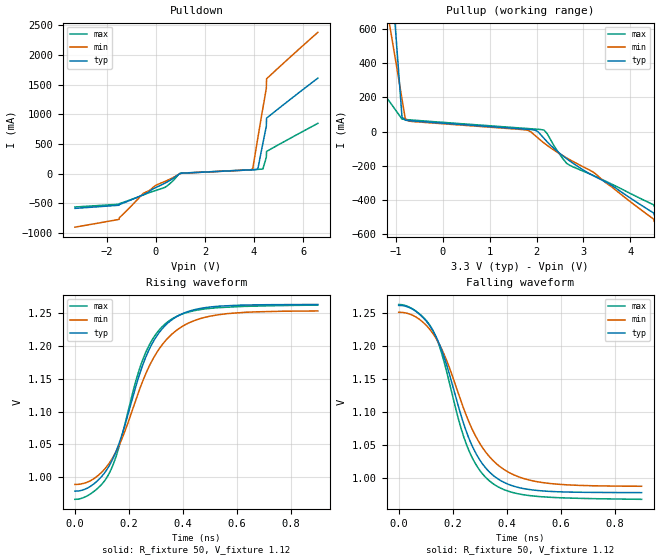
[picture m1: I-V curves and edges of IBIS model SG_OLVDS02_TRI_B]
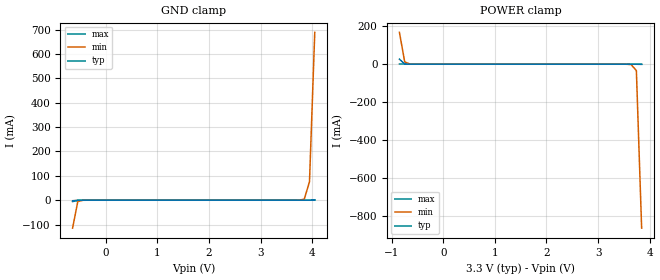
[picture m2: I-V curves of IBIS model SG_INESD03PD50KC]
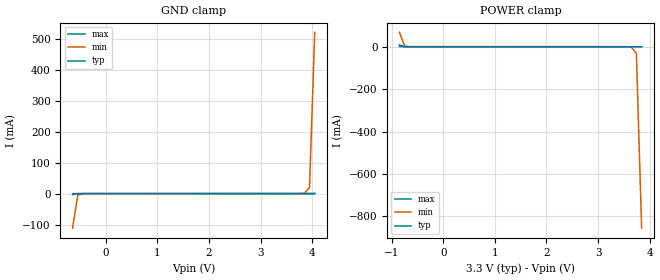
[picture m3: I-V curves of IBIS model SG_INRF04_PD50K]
|   This file is an IBIS representation of the   |
|   Integrated Device Technology, Inc.   |
|   854S54I-02   |
|   DUAL 2:1 AND 1:2, DIFFERENTIAL-TO-LVDS MULTIPLEXER   |
[IBIS Ver]   4.1
[File name]   854s54i_02_3v3.ibs
[File Rev]   1.0
[Date]   16 Apr 2010
[Source]   Originated at Integrated Device Technology, Inc.
[Disclaimer]
IDT hereby grants the user of this IBIS model a non-exclusive,
nontransferable license to use this IBIS model under the following terms.
Before using this IBIS model, the user should read this license.
If the user does not accept these terms,  the IBIS model should be
returned to IDT within 30 days.
   The user is granted this license only to use the IBIS model and
is not granted rights to sell, load, rent, lease or license the IBIS
model in whole or in part, or in modified form to anyone other than
user. User may modify the IBIS model to suit its specific
applications but rights to derivative works and such modifications
shall belong to IDT.
   This IBIS model is provided on an "AS IS" basis and IDT makes
absolutely no warranty with respect to the information contained
herein. IDT DISCLAIMS AND CUSTOMER WAIVES ALL WARRANTIES, EXPRESS
OR IMPLIED, INCLUDING WARRANTIES OF MERCHANTABILITY OR FITNESS FOR
A PARTICULAR PURPOSE. The entire risk as to quality and performance
is with the Customer. ACCORDINGLY, IN NO EVENT SHALL THE COMPANY BE
LIABLE FOR ANY DAMAGES, WHETHER IN CONTRACT OR TORT,INCLUDING ANY
LOST PROFITS OR OTHER INCIDENTAL, CONSEQUENTIAL, EXEMPLARY, OR
PUNITIVE DAMAGES ARISING OUT OF THE USE OR APPLICATION OF THE IBIS
model provided in this package. Further, IDT reserves the right to
make changes without notice to any product herein to improve
reliability, function, or design. IDT does not convey any license
under patent rights or any other intellectual property rights,
including those of third parties.
   IDT is not obligated to provide maintenance or support
for the licensed IBIS model.
[Copyright]   Copyright 2007 by Integrated Device Technology, Inc.
[Component]   854S54KI-02
[Manufacturer] Integrated Device Technology, Inc.
[Package]
|VFQFN 24 Lead
|   typ   min   max
R_pkg   53.3006m   39.9458m   67.5454m
L_pkg   0.925n   0.5704n   1.2967n
C_pkg   0.1079p   0.0821p   0.1352p
[Pin] signal_name  model_name   R_pin   L_pin   C_pin
1   VDD   POWER   67.5454m   1.2967n   0.1352p
2   QA0   SG_OLVDS02_TRI_B   53.7456m   0.9336n   0.1086p
3   nQA0   SG_OLVDS02_TRI_B   39.9458m   0.5704n   0.0821p
4   GND   GND   39.9458m   0.5704n   0.0821p
5   SEL_QB   SG_INESD03PD50KC   53.7456m   0.9336n   0.1086p
6   NC   NC   67.5454m   1.2967n   0.1352p
7   NC   NC   67.5454m   1.2967n   0.1352p
8   INA0   SG_INRF04_PD50K   53.7456m   0.9336n   0.1086p
9   nINA0   SG_INRF04_PMID50   39.9458m   0.5704n   0.0821p
10   INA1   SG_INRF04_PD50K   39.9458m   0.5704n   0.0821p
11   nINA1   SG_INRF04_PMID50   53.7456m   0.9336n   0.1086p
12   NC   NC   67.5454m   1.2967n   0.1352p
13   NC   NC   67.5454m   1.2967n   0.1352p
14   MODE_QAX   SG_INESD03_PD50K   53.7456m   0.9336n   0.1086p
15   GND   GND   39.9458m   0.5704n   0.0821p
16   nQA1   SG_OLVDS02_TRI_B   39.9458m   0.5704n   0.0821p
17   QA1   SG_OLVDS02_TRI_B   53.7456m   0.9336n   0.1086p
18   VDD   POWER   67.5454m   1.2967n   0.1352p
19   NC   NC   67.5454m   1.2967n   0.1352p
20   nINB   SG_INRF04_PD50K   53.7456m   0.9336n   0.1086p
21   INB   SG_INRF04_PMID50   39.9458m   0.5704n   0.0821p
22   nQB   SG_OLVDS02_TRI_B   39.9458m   0.5704n   0.0821p
23   QB   SG_OLVDS02_TRI_B   53.7456m   0.9336n   0.1086p
24   NC   NC   67.5454m   1.2967n   0.1352p
[Diff Pin]  inv_pin  vdiff tdelay_typ tdelay_min  tdelay_max
2   3   NA   0   0   0
8   9   0.15   NA   NA   NA
10   11   0.15   NA   NA   NA
17   16   NA   0   0   0
21   20   0.15   NA   NA   NA
23   22   NA   0   0   0
| Models and submodels in the file (5): SG_OLVDS02_TRI_B (Output), SG_INESD03PD50KC (Input), SG_INRF04_PD50K (Input), SG_INRF04_PMID50 (Input), SG_INESD03_PD50K (Input)
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[Model]   SG_OLVDS02_TRI_B
Model_type   Output
Polarity   Non-Inverting
|   typ   min   max
C_comp   2pF   1.5pF   2.5pF
Vmeas = 1.12V
Rref = 50
Cref = 0
Vref = 1.12V
|   typ   min   max
[Voltage range]   3.3V   3.135V   3.465V
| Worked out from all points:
|   slope of the pulldown table from 0 to 0.495 V, typ, clamps not added: 4.9 ohm
|   slope of the pullup table from 0 to 0.495 V, typ, clamps not added: 49.7 ohm
|   rising waveform, R_fixture 50, V_fixture 1.12: 20-80 % time 141ps typ, 165ps min, 130ps max; typ from 0.979 V to 1.26 V
|   falling waveform, R_fixture 50, V_fixture 1.12: 20-80 % time 141ps typ, 165ps min, 130ps max; typ from 1.26 V to 0.978 V
[Pulldown]
|Voltage   I (typ)   I (min)   I (max)
-3.3V     -582.3mA   -898.2mA   -558.8mA
-1.5V     -529.4mA   -767.2mA   -512.6mA
-1.49V    -518.5mA   -740.2mA   -503.1mA
-526.1mV  -353.6mA   -332.4mA   -359.2mA
369mV     -157.3mA   -129mA     -228.7mA
988.6mV   4.493mA    2.581mA    8.244mA
3.949V    67.95mA    88.23mA    69.88mA
4.156V    82.87mA    606.9mA    74.21mA
4.362V    516.1mA    1.11A      81.89mA
4.5V      797.8mA    1.437A     279.3mA
4.51V     936.5mA    1.598A     376.5mA
6.6V      1.61A      2.38A      848.2mA
[Pullup]
|Voltage   I (typ)   I (min)   I (max)
-3.3V     3.673A     1.802A     451.1mA
-1.5V     2.537A     1.292A     331.3mA
-1.146V   1.096A     645.1mA    179.4mA
-1.008V   595.8mA    420.7mA    126.7mA
-870.3mV  85.62mA    191.8mA    72.93mA
-801.5mV  66.7mA     75.64mA    70.63mA
1.953V    9.214mA    -19.37mA   14.7mA
2.159V    -40.19mA   -67.39mA   8.459mA
2.641V    -159.5mA   -154.7mA   -186.5mA
3.261V    -266.5mA   -248.9mA   -264.5mA
4.51V     -490.6mA   -528.4mA   -439.8mA
6.6V      -547.3mA   -594.3mA   -482.8mA
[Ramp]
|   typ   min   max
dV/dt_r   0.17/0.141n   0.158/0.164n   0.177/0.13n
dV/dt_f   0.17/0.141n   0.158/0.164n   0.177/0.13n
R_load =   50.0000
[Rising Waveform]
R_fixture = 50
V_fixture = 1.12   |Vcc_typ
V_fixture_min = 1.12 |Vcc_min
V_fixture_max = 1.10 |Vcc_max
C_fixture = 0.0p
| Time   typ   min   max
0s        978.8mV    989.1mV    966.4mV
64.86ps   988.2mV    996.5mV    976.7mV
127ps     1.017V     1.021V     1.006V
169.4ps   1.059V     1.054V     1.055V
252.3ps   1.172V     1.148V     1.18V
293.7ps   1.209V     1.183V     1.214V
340.5ps   1.234V     1.21V      1.236V
410.8ps   1.251V     1.233V     1.25V
509.9ps   1.26V      1.246V     1.258V
900ps     1.263V     1.253V     1.262V
[Falling Waveform]
R_fixture = 50
V_fixture = 1.12   |Vcc_typ
V_fixture_min = 1.12 |Vcc_min
V_fixture_max = 1.10 |Vcc_max
C_fixture = 0.0p
| Time   typ   min   max
0s        1.262V     1.252V     1.263V
65.77ps   1.252V     1.244V     1.253V
127ps     1.223V     1.219V     1.224V
170.3ps   1.181V     1.186V     1.173V
250.4ps   1.071V     1.095V     1.052V
291.9ps   1.033V     1.058V     1.017V
339.6ps   1.008V     1.031V     994.4mV
411.7ps   989.5mV    1.008V     979.2mV
508.1ps   981.2mV    994.7mV    972.2mV
900ps     977.8mV    987.4mV    967.6mV
[Model]   SG_INESD03PD50KC
Model_type   Input
Polarity   Non-Inverting
Vinl = 0.8V
Vinh = 2.0V
|   typ   min   max
C_comp   2pF   1.5pF   2.5pF
|   typ   min   max
[Voltage range]  3.3V   3.135V   3.465V
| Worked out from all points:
|   GND clamp passes 1 mA (typ) near -0.55 V on its own axis
|   POWER clamp passes 1 mA (typ) near -0.75 V on its own axis
[GND_clamp]
|Voltage   I(typ)   I(min)   I(max)
-646.4mV  -5.866mA   -114.8mA   -2.202mA
-544.3mV  -860.2uA   -5.306mA   -368.1uA
-442.3mV  -95.82uA   -397.6uA   -22.47uA
3.64V     72.48uA    101uA      67.77uA
3.844V    82.42uA    3.9mA      71.58uA
3.946V    154uA      75.88mA    73.49uA
4.048V    932uA      689.3mA    75.97uA
[POWER_clamp]
|Voltage   I(typ)   I(min)   I(max)
-850.5mV  26.75mA    167.6mA    1.127mA
-748.5mV  932uA      12.37mA    159.1uA
-646.4mV  154uA      763.5uA    81.42uA
3.64V     -10.56uA   -1.878mA   -3.259uA
3.742V    -95.82uA   -33.73mA   -5.166uA
3.844V    -860.2uA   -863.1mA   -8.144uA
[Model]   SG_INRF04_PD50K
Model_type   Input
Polarity   Non-Inverting
Vinl = 0.8V
Vinh = 2.0V
|   typ   min   max
C_comp   2pF   1.5pF   2.5pF
|   typ   min   max
[Voltage range]  3.3V   3.135V   3.465V
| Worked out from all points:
|   GND clamp passes 1 mA (typ) near -0.58 V on its own axis
|   POWER clamp passes 1 mA (typ) near -0.76 V on its own axis
[GND_clamp]
|Voltage   I(typ)   I(min)   I(max)
-646.4mV  -3.138mA   -111.3mA   -21.79uA
-544.3mV  -69.67uA   -4.089mA   -10.18uA
-442.3mV  -9.904uA   -158.5uA   -8.226uA
3.844V    76.6uA     776.7uA    71.58uA
3.946V    81.65uA    19.12mA    73.48uA
4.048V    243.9uA    519.9mA    75.39uA
[POWER_clamp]
|Voltage   I(typ)   I(min)   I(max)
-850.5mV  8.757mA    67.72mA    400uA
-748.5mV  243.9uA    2.557mA    80.45uA
-646.4mV  81.65uA    168.9uA    76.57uA
3.64V     -6.787uA   -1.158mA   -3.258uA
3.742V    -9.904uA   -31.35mA   -5.157uA
3.844V    -69.67uA   -855.7mA   -7.055uA
